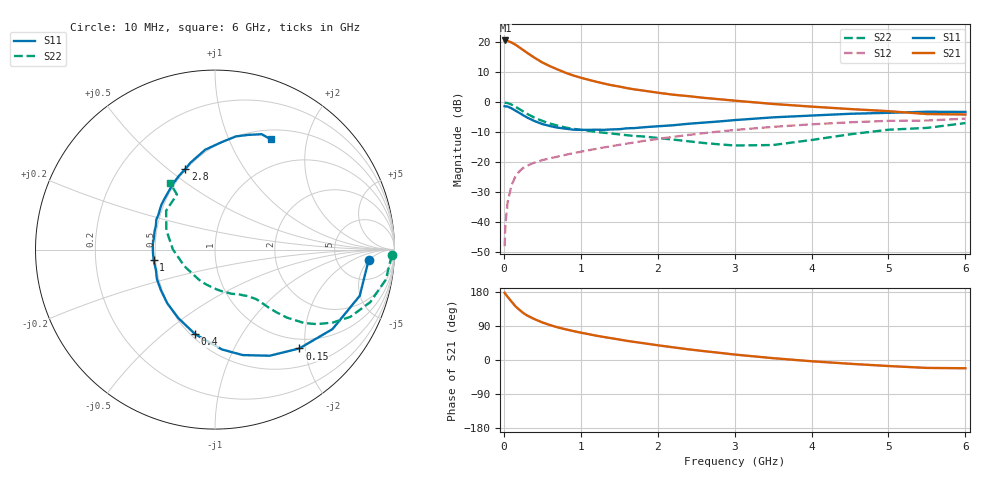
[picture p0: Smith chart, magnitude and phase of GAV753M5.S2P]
! Infineon Technologies  Discrete & RF Semiconductors
! BF775
! Si NPN RF Bipolar Junction Transistor in SOT23
! VCE = 0.75 V  IC = 3.5 mA
! Common Emitter S-Parameters:  May  1996
# GHz  S  MA  R  50
!  f  S11  S21  S12  S22
! GHz  MAG  ANG  MAG  ANG  MAG  ANG  MAG  ANG
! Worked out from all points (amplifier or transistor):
!   36 points, 10 MHz to 6 GHz, reference 50 ohm
!   highest |S21| = 20.6 dB at 20 MHz (marker M1)
!   |S21| within 3 dB of that: start of sweep to 241 MHz
!   unconditionally stable (mu >= 1): 814.6 MHz to end of sweep
!   at 250 MHz: K = 0.42, MSG = 19.7 dB, |S12| = -21.9 dB
!   at 1.4 GHz: K = 1.20, MAG = 7.5 dB, |S12| = -14.7 dB
!   at 6 GHz: K = 1.06, MAG = -0.8 dB, |S12| = -5.5 dB
!   S11 on the Smith chart (normalised r, x): 10 MHz: 11, -5; 150 MHz: 0.82, -1.89; 400 MHz: 0.53, -0.65; 1 GHz: 0.49, -0.06; 2.8 GHz: 0.49, +0.57; 6 GHz: 0.62, +1.44
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0.01  0.858 -3.8  10.58 177.5  0.004 87.2  0.9881 -1.9
0.02  0.8507 -7.2  10.67 174.3  0.009 85.6  0.9779 -4.0
0.05  0.8465 -17.7  10.44 166.5  0.022 80.1  0.9668 -9.9
0.1  0.7903 -34.1  9.869 154.0  0.0416 72.4  0.9131 -18.7
0.15  0.724 -49.5  9.08 141.9  0.0576 63.7  0.8422 -26.4
0.2  0.6654 -62.7  8.211 132.8  0.0702 58.6  0.7715 -31.8
0.25  0.6079 -75.2  7.418 124.4  0.0799 54.1  0.7032 -36.2
0.3  0.5578 -86.0  6.685 117.7  0.0875 51.3  0.6429 -39.5
0.4  0.4839 -103.2  5.491 107.7  0.0986 47.7  0.5512 -43.4
0.5  0.4329 -118.2  4.59 99.2  0.1084 46.0  0.488 -45.6
0.6  0.4001 -131.7  3.978 92.2  0.1162 45.4  0.4407 -47.2
0.7  0.3766 -143.2  3.502 86.2  0.1242 45.5  0.4061 -48.3
0.8  0.3629 -153.2  3.102 81.1  0.1327 45.5  0.3792 -49.3
1  0.3469 -170.3  2.558 72.2  0.1496 45.7  0.3464 -51.4
1.1  0.3462 -177.5  2.365 68.3  0.1582 46.0  0.3334 -53.0
1.6  0.3672 152.9  1.715 50.6  0.2046 45.5  0.2818 -62.0
2.2  0.4129 129.1  1.334 33.5  0.2646 42.1  0.2386 -79.1
2.8  0.4779 110.3  1.121 19.0  0.3246 36.2  0.1987 -106.0
3.5  0.5591 95.6  0.935 4.8  0.3884 27.6  0.1936 -151.0
4.5  0.6411 79.6  0.769 -10.0  0.4626 14.7  0.292 158.2
5.5  0.6935 68.0  0.635 -20.9  0.4949 1.1  0.3734 124.6
6  0.6886 63.2  0.624 -21.8  0.5324 -2.7  0.4489 124.0
